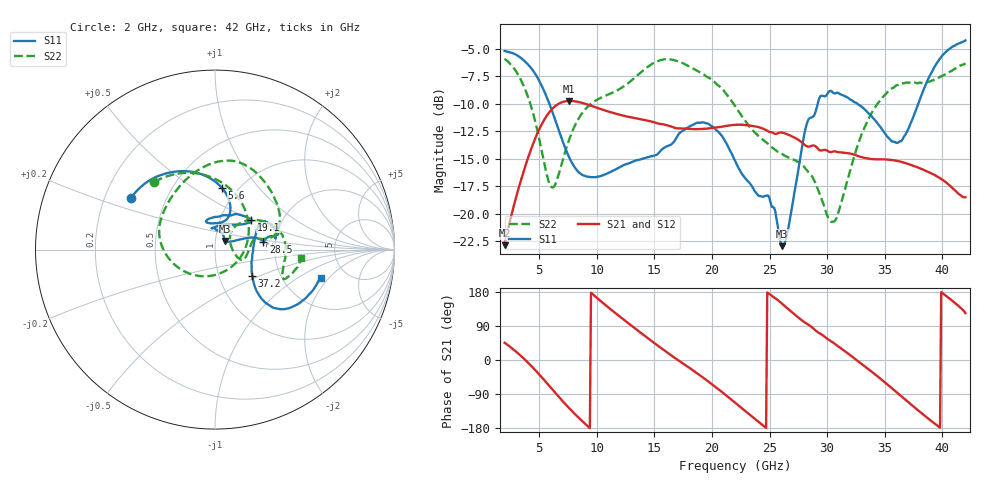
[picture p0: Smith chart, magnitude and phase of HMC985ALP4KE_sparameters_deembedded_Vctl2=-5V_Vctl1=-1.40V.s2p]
!s2p File: Measurements: S11, S21, S12, S22
# GHz S dB R 50.0
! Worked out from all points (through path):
!   401 points, 2 GHz to 42 GHz, reference 50 ohm
!   highest |S21| = -9.74 dB at 7.6 GHz (marker M1); lowest = -22.8 dB at 2 GHz (marker M2)
!   lowest |S11| = -22.9 dB at 26.1 GHz (marker M3), VSWR 1.15, Z = 55.3 + j5.3 ohm
!   |S11| at or under -10 dB: 5.889 GHz to 29.17 GHz (23.28 GHz wide, 133 % of centre); 32.64 GHz to 37.9 GHz (5.264 GHz wide, 14.9 % of centre)
!   |S22| runs from -20.7 to -5.9 dB; largest |S21 - S12| = 0.00031
!   S11 on the Smith chart (normalised r, x): 2 GHz: 0.31, +0.26; 5.6 GHz: 0.85, +0.66; 19.1 GHz: 1.40, +0.50; 28.5 GHz: 1.73, +0.16; 37.2 GHz: 1.44, -0.45; 42 GHz: 3.24, -1.67
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2  -5.19 148.2  -22.84 45.5  -22.85 45.5  -5.91 131.9
3.6  -5.99 121.7  -16.32 5.7  -16.32 5.7  -8.24 87.8
4.7  -7.35 100.7  -13.04 -27.9  -13.04 -27.9  -11.78 45.8
5.6  -9.25 83.4  -11.17 -58.7  -11.18 -58.6  -16.16 -9.0
6.3  -11.18 72.8  -10.29 -83.3  -10.30 -83.3  -17.50 -71.5
7.6  -14.86 68.9  -9.74 -127.0  -9.74 -127.0  -13.25 -148.8
8.7  -16.43 80.8  -9.90 -160.2  -9.91 -160.2  -10.90 -178.9
10.1  -16.62 97.2  -10.39 161.7  -10.39 161.7  -9.58 159.5
12.1  -15.71 107.7  -11.02 112.2  -11.03 112.2  -8.58 133.4
15.4  -14.44 80.7  -11.81 35.7  -11.81 35.7  -6.08 84.6
19.1  -11.70 39.8  -12.29 -43.6  -12.29 -43.6  -7.25 39.1
22  -15.16 52.7  -11.91 -112.5  -11.91 -112.4  -10.20 11.9
24.9  -18.36 94.0  -12.52 176.1  -12.52 176.1  -13.68 10.2
26.1  -22.93 41.9  -12.62 148.1  -12.62 148.1  -14.57 -2.5
28.5  -11.29 9.1  -13.87 90.7  -13.88 90.7  -16.38 -21.3
28.7  -11.22 8.5  -13.80 86.0  -13.80 86.1  -16.61 -20.9
30.6  -9.04 15.0  -14.31 44.1  -14.32 44.1  -20.68 21.8
33.2  -10.45 31.0  -14.90 -15.3  -14.91 -15.3  -12.26 41.8
35.4  -13.17 8.5  -15.08 -68.9  -15.08 -68.9  -8.80 19.0
37.2  -11.90 -35.1  -15.53 -115.2  -15.53 -115.1  -8.06 -1.1
39.7  -6.02 -41.7  -16.68 -176.3  -16.68 -176.3  -7.62 -23.4
42  -4.24 -15.2  -18.48 123.9  -18.49 123.9  -6.31 -5.8
